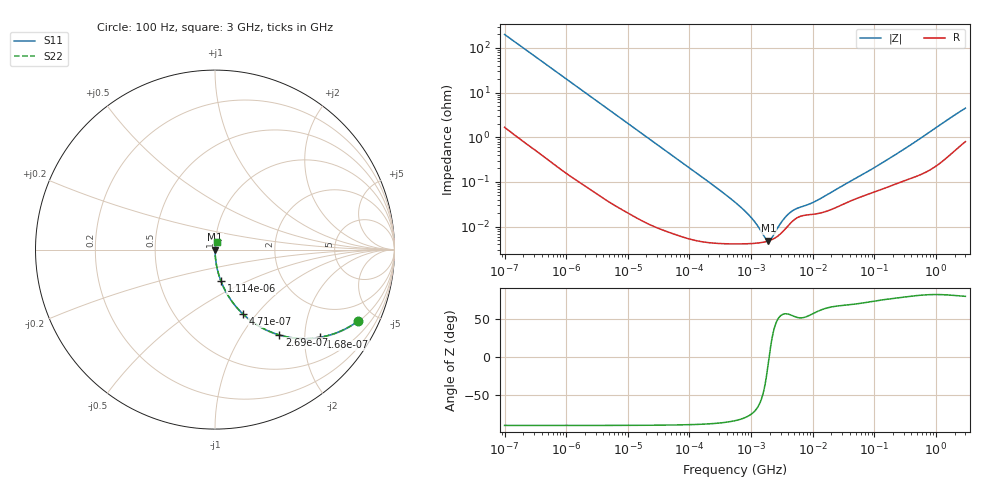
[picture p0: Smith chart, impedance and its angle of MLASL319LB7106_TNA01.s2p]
! MLASL319LB7106_TNA01  S-PARAMETER MODEL  ( Standard Model )
! Model Generated by TAIYO YUDEN Corporation (http://www.ty-top.com)
! Version 1.0
! TAIYO YUDEN Control No. 220601
! Copyright(c) 2011 TAIYO YUDEN CO.,LTD. All Rights Reserved.
! Product Description (link to TY-COMPAS)
! https://ds.yuden.co.jp/TYCOMPAS/or/detail?pn=MLASL319LB7106MTNA01&u=M
! Products Name : Multilayer Ceramic Capacitors
! Characteristics :
!  Capacitance : 10 [uF] , Rated Voltage : 10 [V] , TCC : X7R
!  Case Size : 3.2 x 1.6 / 0.126 x 0.063 [mm/inch] , Thickness : 0.85 / 0.033 [mm/inch]
!  (Conditions: Temperature = 25 [degC] , DC Bias Voltage = 0 [V])
! External Node Assignments :
!  1  o---| |---o  2
! GND o---------o GND
! Frequency Range : 100Hz  -  3GHz  [ 401 STEP ]
# MHZ S RI R 50
! Freq[MHz].  S11 Real  S11 Imag  S21 Real  S21 Imag  S12 Real  S12 Imag  S22 Real  S22 Imag
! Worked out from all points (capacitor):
!   401 points, 100 Hz to 3 GHz, reference 50 ohm
!   read as one part in series: C = 7.97 uF near 109 Hz
!   lowest |Z| = 4.82 mohm at 1.908 MHz (marker M1)
!   series resonance near 1.961 MHz, so ESL is about 830 pH
!   S11 on the Smith chart (normalised r, x): 100 Hz: 1.03, -3.99; 168 Hz: 1.02, -2.39; 269 Hz: 1.01, -1.49; 471 Hz: 1.01, -0.85; 1.114 kHz: 1.00, -0.36; 3 GHz: 1.02, +0.09
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0.0001  0.7973 -0.3978  0.2027 0.3978  0.2027 0.3978  0.7973 -0.3978
0.000119  0.7371 -0.4361  0.2629 0.4361  0.2629 0.4361  0.7371 -0.4361
0.000168  0.587 -0.4883  0.413 0.4883  0.413 0.4883  0.587 -0.4883
0.000269  0.3583 -0.4755  0.6417 0.4755  0.6417 0.4755  0.3583 -0.4755
0.000471  0.1563 -0.3592  0.8437 0.3592  0.8437 0.3592  0.1563 -0.3592
0.000694  0.0796 -0.2668  0.9204 0.2668  0.9204 0.2668  0.0796 -0.2668
0.001114  0.0331 -0.1751  0.9669 0.1751  0.9669 0.1751  0.0331 -0.1751
0.001788  0.0135 -0.1116  0.9865 0.1116  0.9865 0.1116  0.0135 -0.1116
0.005476  0.0017 -0.0371  0.9983 0.0371  0.9983 0.0371  0.0017 -0.0371
0.031977  0.000132 -0.00642  0.9999 0.00642  0.9999 0.00642  0.000132 -0.00642
0.221826  4.41e-05 -0.000923  1 0.000923  1 0.000923  4.41e-05 -0.000923
0.547723  4.11e-05 -0.00035  1 0.00035  1 0.00035  4.11e-05 -0.00035
0.842342  4.14e-05 -0.000202  1 0.000202  1 0.000202  4.14e-05 -0.000202
1.295438  4.3e-05 -9.16e-05  1 9.16e-05  1 9.16e-05  4.3e-05 -9.16e-05
1.411895  4.37e-05 -7.2e-05  1 7.2e-05  1 7.2e-05  4.37e-05 -7.2e-05
1.908323  4.79e-05 -5.85e-06  1 5.85e-06  1 5.85e-06  4.79e-05 -5.85e-06
2.69274  6.1e-05 7.08e-05  0.9999 -7.08e-05  0.9999 -7.08e-05  6.1e-05 7.08e-05
3.79959  9.7e-05 0.000148  0.9999 -0.000148  0.9999 -0.000148  9.7e-05 0.000148
4.711951  0.000133 0.000184  0.9999 -0.000184  0.9999 -0.000184  0.000133 0.000184
9.794414  0.000188 0.000284  0.9998 -0.000284  0.9998 -0.000284  0.000188 0.000284
175.1444  0.000805 0.00326  0.9992 -0.00326  0.9992 -0.00326  0.000805 0.00326
3000  0.0098 0.0432  0.9902 -0.0432  0.9902 -0.0432  0.0098 0.0432
